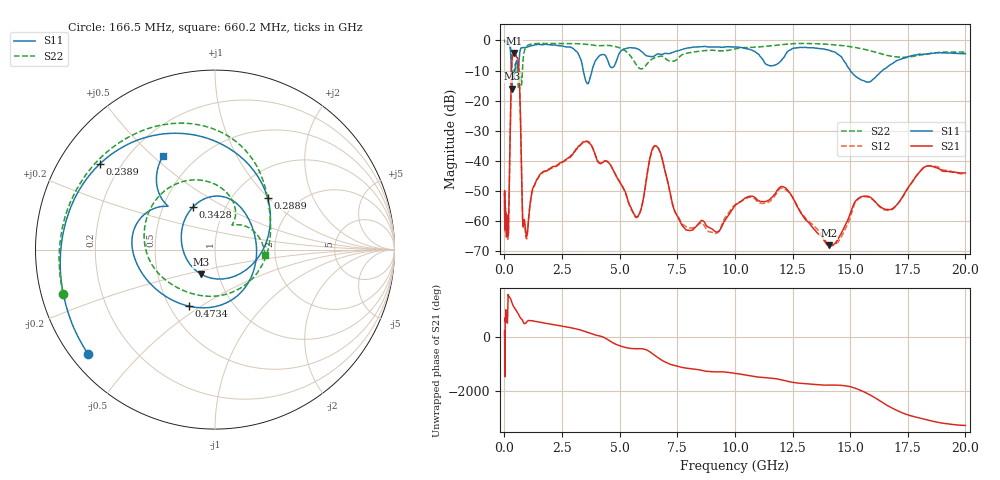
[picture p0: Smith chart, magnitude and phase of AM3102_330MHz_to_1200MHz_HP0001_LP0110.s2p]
! Date/Time: Tue, Sep 11, 2018 5:09 PM
! Network Analyzer: Agilent Technologies E8362B Rev: A.07.50.63
! Sweep from 0.010 to 20.000 GHz, 1601 Points, Sweep Type: LOG
! Power Supply: 4.950 V, 0.001 A
# Hz S DB R 50
!freq MagS11 AngS11 MagS21 AngS21 MagS12 AngS12 MagS22 AngS22
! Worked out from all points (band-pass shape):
!   1601 points, 10 MHz to 20 GHz, reference 50 ohm
!   highest |S21| = -4.16 dB at 416.5 MHz (marker M1); lowest = -68.2 dB at 14.07 GHz (marker M2)
!   |S21| within 3 dB of the highest: 323.5 MHz to 607.1 MHz (283.7 MHz wide, 61 % of centre)
!   lowest |S11| = -16.1 dB at 316.2 MHz (marker M3), VSWR 1.37, Z = 41.5 - j11.8 ohm
!   |S11| at or under -10 dB: 295.4 MHz to 457.4 MHz (162 MHz wide, 43 % of centre); 3.421 GHz to 3.802 GHz (380.8 MHz wide, 10.5 % of centre); 15.01 GHz to 16.4 GHz (1.393 GHz wide, 8.87 % of centre)
!   |S22| runs from -15.6 to -0.2 dB; largest |S21 - S12| = 0.01
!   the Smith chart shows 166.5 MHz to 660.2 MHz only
!   S11 on the Smith chart (normalised r, x): 166.5 MHz: 0.05, -0.36; 238.9 MHz: 0.12, +0.33; 288.9 MHz: 1.42, +0.99; 342.8 MHz: 0.71, +0.36; 473.4 MHz: 0.62, -0.45; 660.2 MHz: 0.33, +0.54
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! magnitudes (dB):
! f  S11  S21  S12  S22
! 10 MHz  0.0  -57.4  -51.8  -0.2
! 35.55 MHz  0.0  -59.9  -60.0  -0.4
! 126.4 MHz  -0.4  -62.3  -64.7  -0.9
! 166.5 MHz  -0.8  -64.8  -64.6  -1.1
! 238.9 MHz  -1.9  -36.8  -36.8  -1.8
! 288.9 MHz  -7.7  -15.2  -15.3  -3.8
! 316.2 MHz  -16.1  -8.1  -8.1  -7.3
! 342.8 MHz  -11.4  -5.7  -5.8  -10.2
! 416.5 MHz  -12.6  -4.2  -4.2  -10.3
! 447.2 MHz  -10.6  -4.3  -4.4  -8.7
! 473.4 MHz  -9.2  -4.6  -4.6  -7.9
! 660.2 MHz  -4.5  -15.1  -15.2  -11.1
! 817.6 MHz  -2.4  -61.9  -62.4  -6.0
! 1.59 GHz  -1.4  -44.2  -44.3  -1.0
! 3.599 GHz  -14.3  -33.7  -33.5  -1.3
! 5.652 GHz  -2.5  -58.1  -58.4  -7.2
! 6.58 GHz  -4.7  -35.1  -35.2  -5.6
! 7.882 GHz  -2.6  -63.1  -61.9  -4.3
! 12.03 GHz  -6.4  -48.6  -49.1  -1.4
! 14.07 GHz  -3.2  -68.2  -68.3  -1.3
! 15.7 GHz  -13.8  -51.8  -52.0  -3.1
! 20 GHz  -4.4  -44.1  -44.6  -3.9
